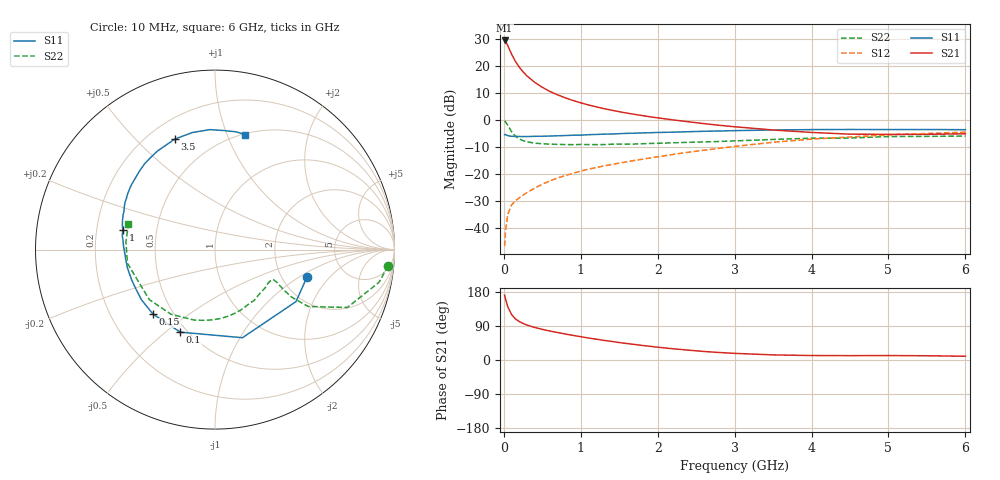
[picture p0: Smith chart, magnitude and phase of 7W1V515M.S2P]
! Infineon Technologies  Discrete & RF Semiconductors
! BFS17W
! Si NPN RF Bipolar Junction Transistor in SOT323
! VCE = 1.5 V  IC = 15 mA
! Common Emitter S-Parameters:  August  1999
# GHz  S  MA  R  50
!  f  S11  S21  S12  S22
! GHz  MAG  ANG  MAG  ANG  MAG  ANG  MAG  ANG
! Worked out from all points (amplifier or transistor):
!   36 points, 10 MHz to 6 GHz, reference 50 ohm
!   highest |S21| = 29.6 dB at 10 MHz (marker M1)
!   |S21| within 3 dB of that: start of sweep to 67.92 MHz
!   unconditionally stable (mu >= 1): 274.7 MHz to end of sweep
!   at 250 MHz: K = 0.96, MSG = 22.9 dB, |S12| = -27.9 dB
!   at 1.4 GHz: K = 1.26, MAG = 7.0 dB, |S12| = -16.6 dB
!   at 6 GHz: K = 1.10, MAG = -2.2 dB, |S12| = -4.5 dB
!   S11 on the Smith chart (normalised r, x): 10 MHz: 2.74, -1.17; 100 MHz: 0.46, -0.56; 150 MHz: 0.39, -0.37; 1 GHz: 0.31, +0.09; 3.5 GHz: 0.30, +0.65; 6 GHz: 0.51, +1.16
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0.01  0.5347 -16.6  30.34 171.5  0.0045 80.3  0.9692 -5.3
0.02  0.5363 -32.7  29.5 162.5  0.0081 81.0  0.9316 -11.3
0.05  0.5142 -72.7  24.53 141.0  0.0174 65.9  0.8049 -23.6
0.1  0.4989 -112.8  16.93 120.1  0.0263 53.6  0.6088 -31.4
0.15  0.4985 -133.9  12.41 108.6  0.0316 52.9  0.5026 -31.8
0.2  0.496 -145.8  9.695 101.5  0.0356 54.7  0.4476 -30.5
0.25  0.4923 -154.1  7.901 96.4  0.0401 55.4  0.4138 -29.1
0.3  0.4941 -159.9  6.655 92.3  0.0448 58.5  0.3954 -28.1
0.4  0.4987 -168.5  5.058 85.9  0.054 60.9  0.372 -27.3
0.5  0.5005 -174.2  4.076 80.9  0.0642 63.2  0.3629 -27.4
0.6  0.5045 -178.8  3.403 76.4  0.0738 64.1  0.3566 -28.4
0.8  0.5158 173.9  2.59 68.5  0.0928 65.4  0.3502 -32.4
1  0.5249 168.1  2.095 61.5  0.1124 66.0  0.3517 -37.0
1.1  0.5344 165.0  1.913 58.0  0.1221 66.0  0.35 -40.3
1.3  0.5473 159.3  1.637 51.8  0.1402 66.0  0.3503 -46.7
1.6  0.5665 152.1  1.347 43.5  0.1676 65.6  0.3557 -56.6
2.2  0.5961 138.3  1.008 29.6  0.2295 64.3  0.3778 -78.0
2.8  0.6265 124.7  0.8 19.8  0.2984 60.6  0.3998 -99.8
3.5  0.6551 110.1  0.654 13.5  0.3862 53.8  0.4358 -124.4
4.5  0.6691 92.5  0.547 11.5  0.4843 40.9  0.4637 -158.2
5.5  0.6667 80.0  0.543 11.2  0.5631 29.1  0.4981 175.1
6  0.6625 75.3  0.556 9.9  0.5953 23.5  0.5031 163.4
